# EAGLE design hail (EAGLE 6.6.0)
AUTHOR: Branden Ghena; REV: B; TITLE: Hail

## Sheet 1 of 4: Microcontroller
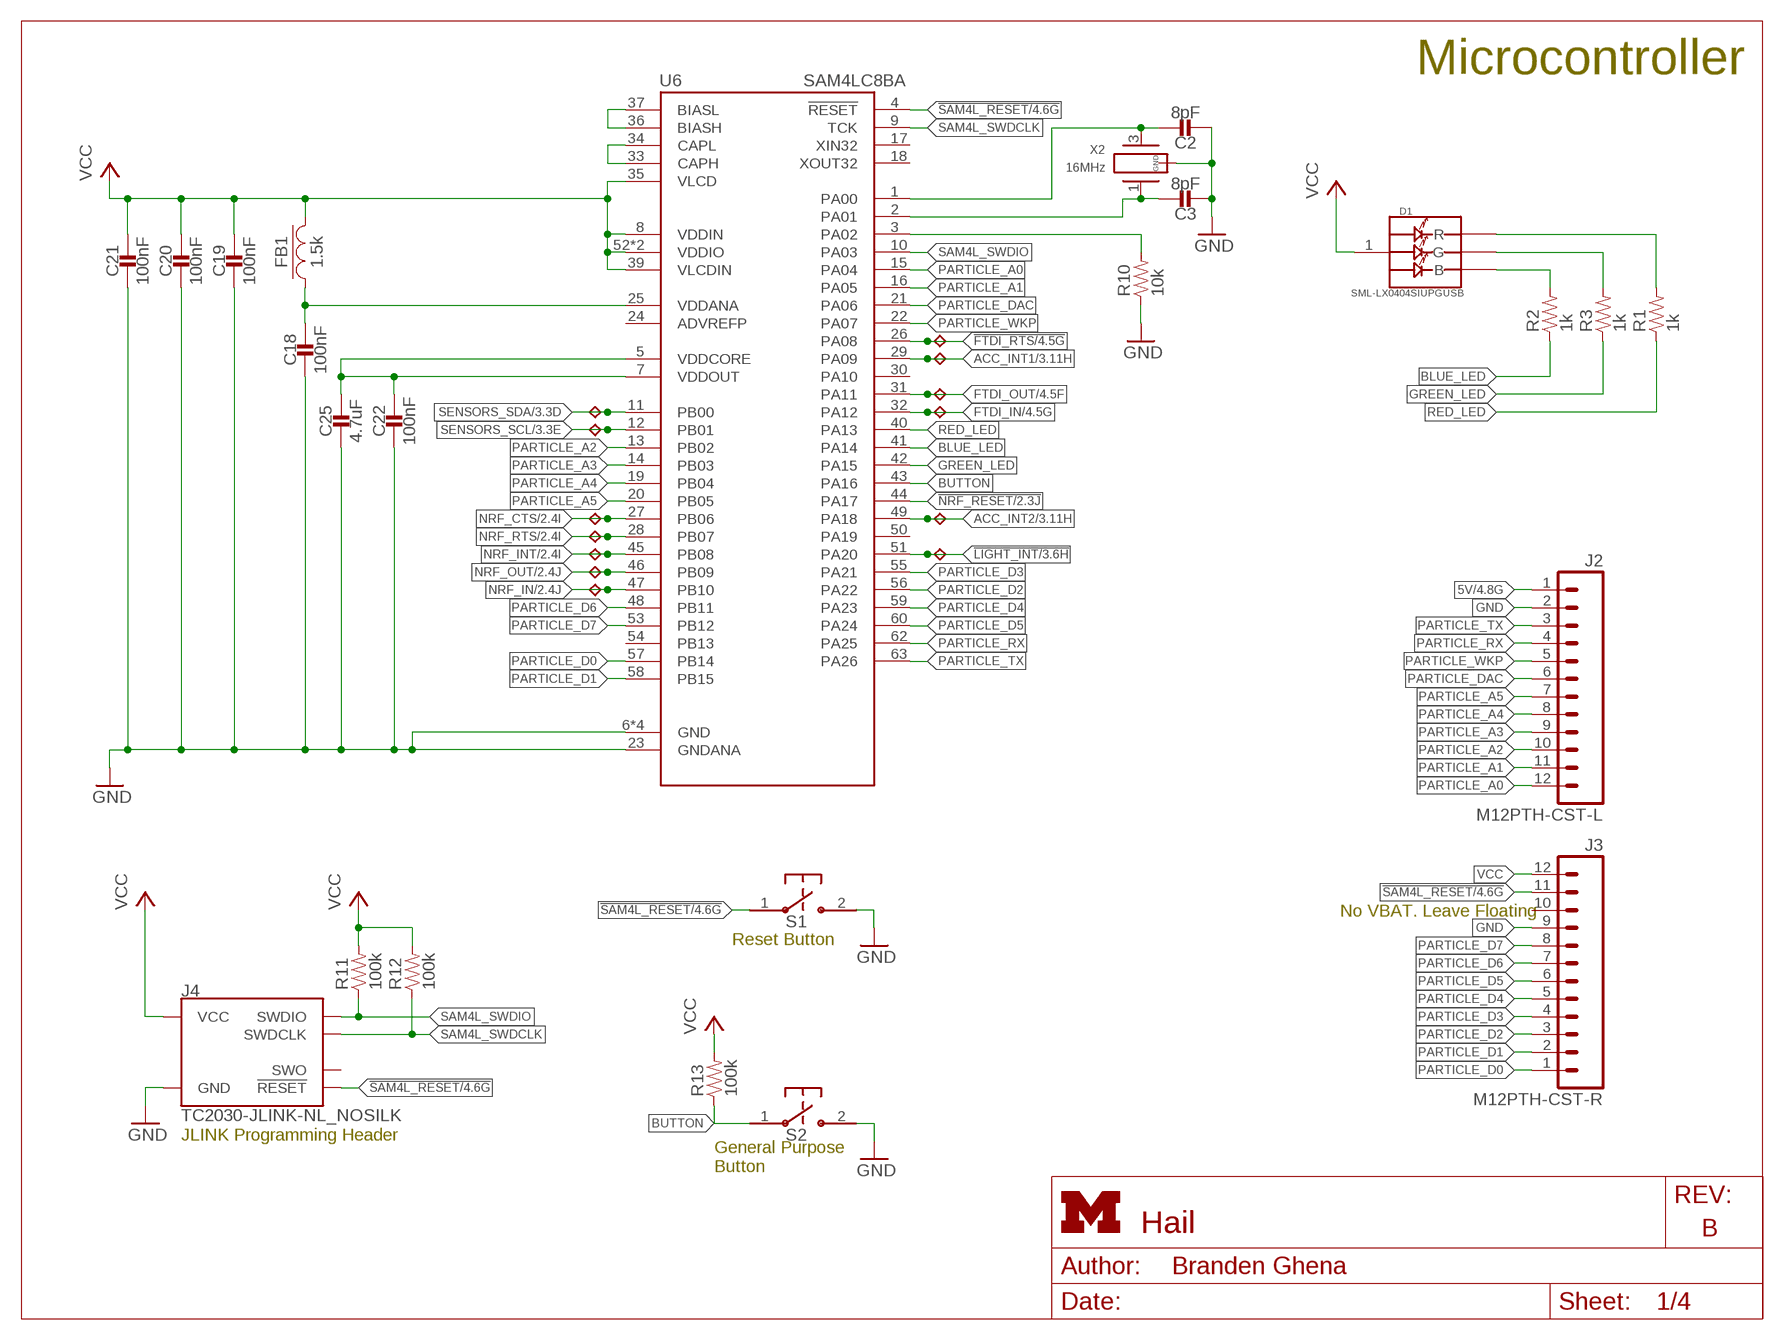
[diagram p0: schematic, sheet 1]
FRAME4 (LETTER_L_UMICH): HEIGHT: 8.5in; WIDTH: 11in
FRAME5 (LETTER_L_UMICH): HEIGHT: 8.5in; WIDTH: 11in

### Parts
C2  8pF  CAPACITOR0402_CAP  [0402_CAP]
C3  8pF  CAPACITOR0402_CAP  [0402_CAP]
C18  100nF  CAPACITOR0402_CAP  [0402_CAP]
C19  100nF  CAPACITOR0402_CAP  [0402_CAP]
C20  100nF  CAPACITOR0402_CAP  [0402_CAP]
C21  100nF  CAPACITOR0402_CAP  [0402_CAP]
C22  100nF  CAPACITOR0402_CAP  [0402_CAP]
C25  4.7uF  CAPACITOR0402_CAP  [0402_CAP]
D1  SML-LX0404SIUPGUSB  [1MM_SQ_4PAD]
FB1  1.5k  FERRITE_BEAD0402  [0402_CAP]
J2  M12PTH-CST-L  [1X12-CASTELLATED]
J3  M12PTH-CST-R  [1X12-CASTELLATED]
J4  TC2030-JLINK-NL_NOSILK  [TC2030-IDC-NL_NOSILK]
R1  1k  RESISTOR0402_RES  [0402_RES]
R2  1k  RESISTOR0402_RES  [0402_RES]
R3  1k  RESISTOR0402_RES  [0402_RES]
R10  10k  RESISTOR0402_RES  [0402_RES]
R11  100k  RESISTOR0402_RES  [0402_RES]
R12  100k  RESISTOR0402_RES  [0402_RES]
R13  100k  RESISTOR0402_RES  [0402_RES]
S1  B3U-1000P  [B3U-1000P]
S2  B3U-1000P  [B3U-1000P]
TP1  TPB1,27  [B1,27]
TP2  TPB1,27  [B1,27]
TP3  TPB1,27  [B1,27]
TP4  TPB1,27  [B1,27]
TP5  TPB1,27  [B1,27]
TP6  TPB1,27  [B1,27]
TP7  TPB1,27  [B1,27]
TP8  TPB1,27  [B1,27]
TP9  TPB1,27  [B1,27]
TP10  TPB1,27  [B1,27]
TP11  TPB1,27  [B1,27]
TP12  TPB1,27  [B1,27]
TP13  TPB1,27  [B1,27]
U6  SAM4LC8BA  [QFN-64-9MM]
X2  16MHz  FH1600015  [FHXXX]

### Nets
5V: J2.1 ; also sheet 4
!FTDI_RTS: TP11.TP U6.26(PA08) ; also sheet 4
!LIGHT_INT: TP10.TP U6.51(PA20) ; also sheet 3
!NRF_RESET: U6.44(PA17) ; also sheet 2
!SAM4L_RESET: J3.11 J4.3(!RESET) S1.1 U6.4(!RESET) ; also sheet 4
ACC_INT1: TP8.TP U6.29(PA09) ; also sheet 3
ACC_INT2: TP9.TP U6.49(PA18) ; also sheet 3
BLUE_LED: R2.1 U6.41(PA14)
BUCK/LDO_N1: R10.2 U6.3(PA02)
BUTTON: R13.1 S2.1 U6.43(PA16)
FTDI_IN: TP13.TP U6.32(PA12) ; also sheet 4
FTDI_OUT: TP12.TP U6.31(PA11) ; also sheet 4
GND: C2.2 C3.2 C18.2 C19.2 C20.2 C21.2 C22.2 C25.2 J2.2 J3.9 J4.5(GND) R10.1 S1.2 S2.2 U6.6(GND) U6.23(GNDANA) U6.38(GND) U6.64(GND) U6.GND X2.2(GND) X2.4(GND) ; also sheet 2,3,4
GREEN_LED: R3.1 U6.42(PA15)
N$7: D1.3(B) R2.2
N$8: D1.4(G) R3.2
N$9: D1.2(R) R1.2
N$15: U6.36(BIASH) U6.37(BIASL)
N$18: U6.33(CAPH) U6.34(CAPL)
N$20: C18.1 FB1.1 U6.25(VDDANA)
N$22: C22.1 C25.1 U6.5(VDDCORE) U6.7(VDDOUT)
NRF_CTS: TP1.TP U6.27(PB06) ; also sheet 2
NRF_IN: TP5.TP U6.47(PB10) ; also sheet 2
NRF_INT: TP3.TP U6.45(PB08) ; also sheet 2
NRF_OUT: TP4.TP U6.46(PB09) ; also sheet 2
NRF_RTS: TP2.TP U6.28(PB07) ; also sheet 2
PARTICLE_A0: J2.12 U6.15(PA04)
PARTICLE_A1: J2.11 U6.16(PA05)
PARTICLE_A2: J2.10 U6.13(PB02)
PARTICLE_A3: J2.9 U6.14(PB03)
PARTICLE_A4: J2.8 U6.19(PB04)
PARTICLE_A5: J2.7 U6.20(PB05)
PARTICLE_D0: J3.1 U6.57(PB14)
PARTICLE_D1: J3.2 U6.58(PB15)
PARTICLE_D2: J3.3 U6.56(PA22)
PARTICLE_D3: J3.4 U6.55(PA21)
PARTICLE_D4: J3.5 U6.59(PA23)
PARTICLE_D5: J3.6 U6.60(PA24)
PARTICLE_D6: J3.7 U6.48(PB11)
PARTICLE_D7: J3.8 U6.53(PB12)
PARTICLE_DAC: J2.6 U6.21(PA06)
PARTICLE_RX: J2.4 U6.62(PA25)
PARTICLE_TX: J2.3 U6.63(PA26)
PARTICLE_WKP: J2.5 U6.22(PA07)
RED_LED: R1.1 U6.40(PA13)
SAM4L_SWDCLK: J4.4(SWDCLK) R12.1 U6.9(TCK)
SAM4L_SWDIO: J4.2(SWDIO) R11.1 U6.10(PA03)
SAM4L_XIN1: C2.1 U6.1(PA00) X2.3
SAM4L_XOUT1: C3.1 U6.2(PA01) X2.1
SENSORS_SCL: TP7.TP U6.12(PB01) ; also sheet 3
SENSORS_SDA: TP6.TP U6.11(PB00) ; also sheet 3
VCC: C19.1 C20.1 C21.1 D1.1(VDD) FB1.2 J3.12 J4.1(VCC) R11.2 R12.2 R13.2 U6.8(VDDIN) U6.35(VLCD) U6.39(VLCDIN) U6.52(VDDIO) U6.61(VDDIO) ; also sheet 2,3,4
Unconnected: J3.10 J4.6(SWO) U6.17(XIN32) U6.18(XOUT32) U6.30(PA10) U6.50(PA19) U6.54(PB13)

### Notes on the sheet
- Microcontroller
- No VBAT. Leave Floating
- Reset Button
- JLINK Programming Header
- General Purpose
  Button

## Sheet 2 of 4: BLE Radio
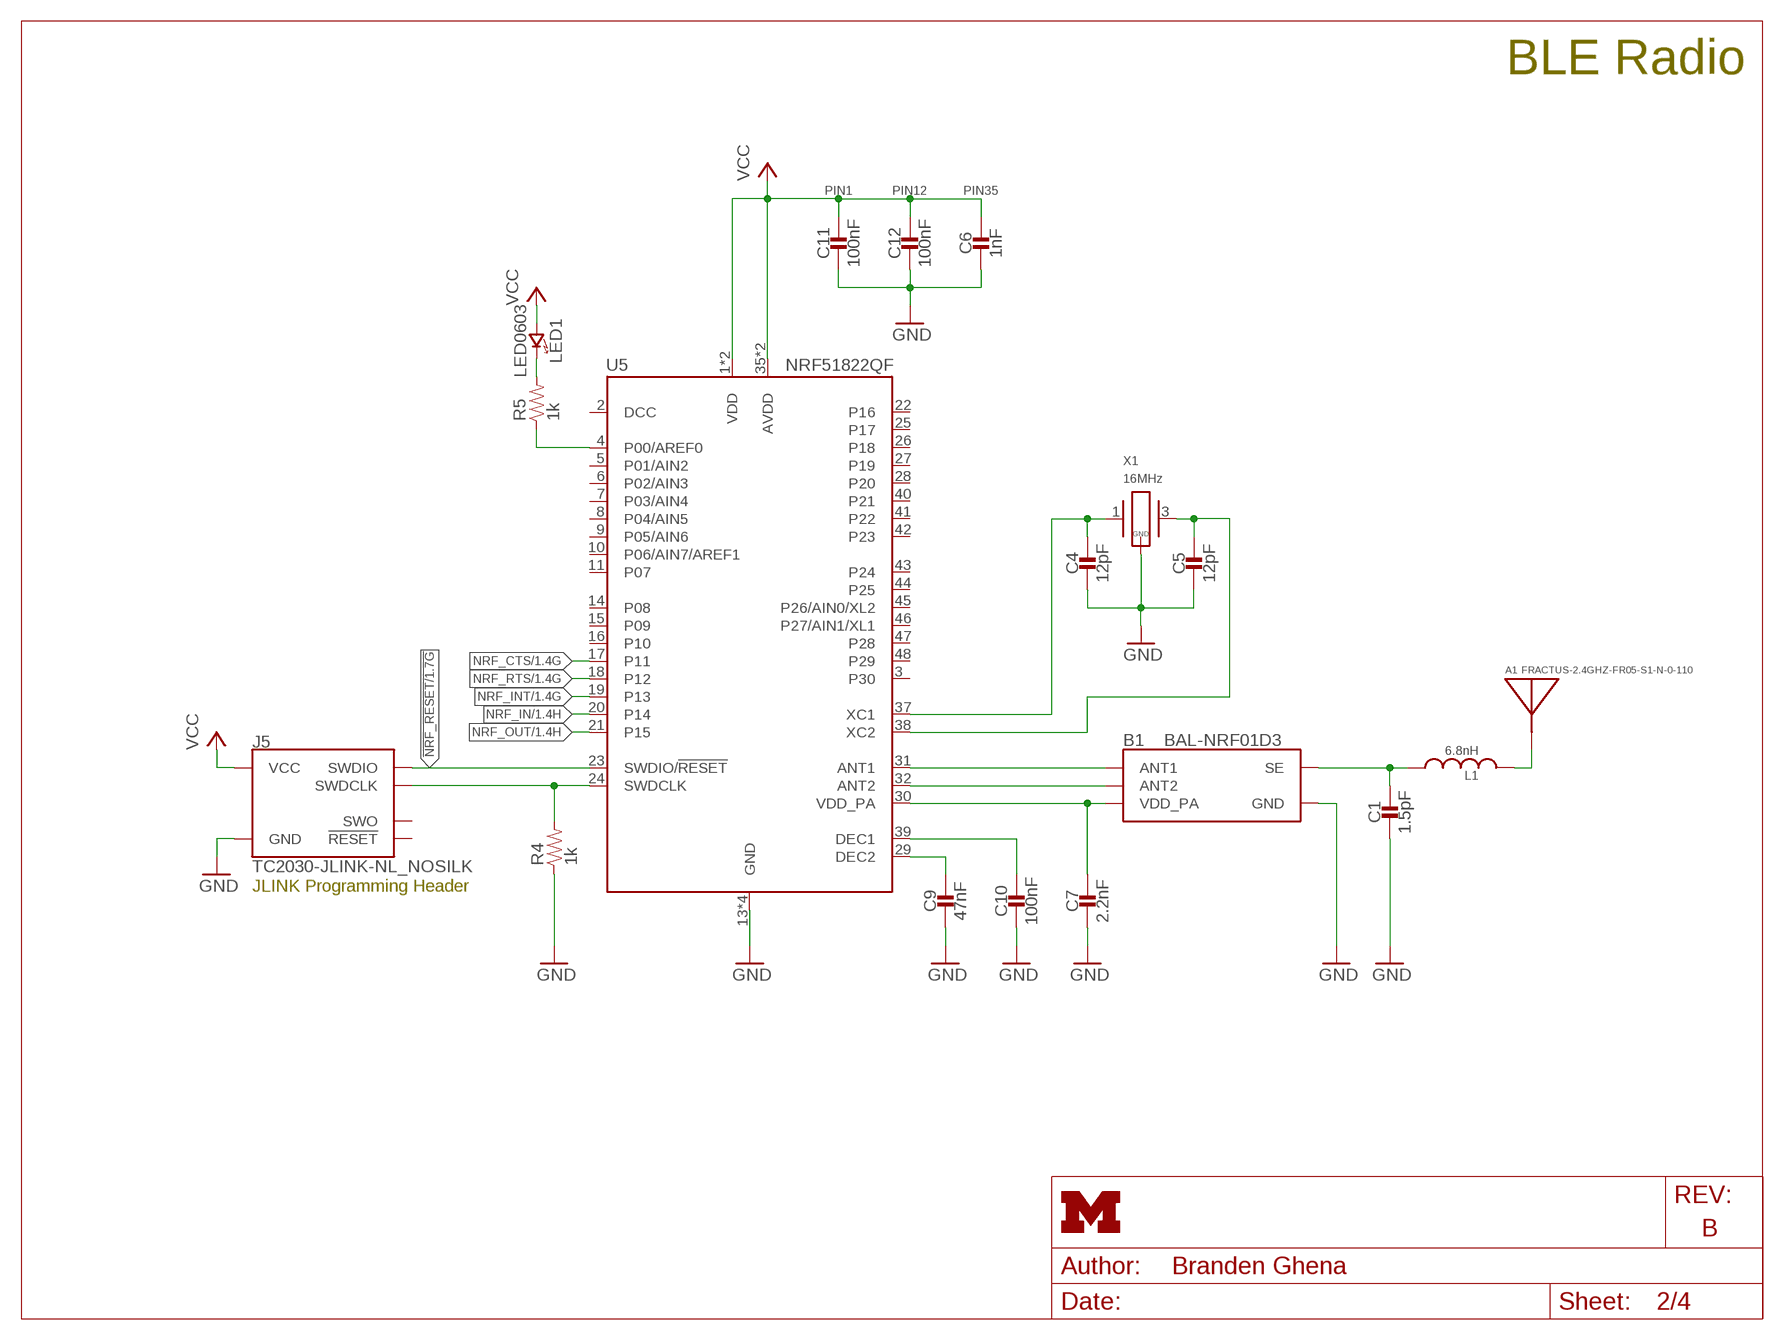
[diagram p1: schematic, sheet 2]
FRAME2 (LETTER_L_UMICH): HEIGHT: 8.5in; WIDTH: 11in
FRAME3 (LETTER_L_UMICH): HEIGHT: 8.5in; TITLE: Hail; WIDTH: 11in

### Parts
A1  FRACTUS-2.4GHZ-FR05-S1-N-0-110  [FRACTUS-ANTENNA-FR05-S1-N-0-110]
B1  BAL-NRF01D3  [BAL-NRF01D3]
C1  1.5pF  CAPACITOR0402_CAP  [0402_CAP]
C4  12pF  CAPACITOR0402_CAP  [0402_CAP]
C5  12pF  CAPACITOR0402_CAP  [0402_CAP]
C6  1nF  CAPACITOR0402_CAP  [0402_CAP]
C7  2.2nF  CAPACITOR0402_CAP  [0402_CAP]
C9  47nF  CAPACITOR0402_CAP  [0402_CAP]
C10  100nF  CAPACITOR0402_CAP  [0402_CAP]
C11  100nF  CAPACITOR0402_CAP  [0402_CAP]
C12  100nF  CAPACITOR0402_CAP  [0402_CAP]
J5  TC2030-JLINK-NL_NOSILK  [TC2030-IDC-NL_NOSILK]
L1  6.8nH  INDUCTOR0402  [0402_CAP]
LED1  LED0603  [LED-0603]
R4  1k  RESISTOR0402_RES  [0402_RES]
R5  1k  RESISTOR0402_RES  [0402_RES]
U5  NRF51822QF  [QFN-48-6MM]
X1  16MHz  TXC-8Y  [TXC-8Y]

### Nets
!NRF_RESET: J5.2(SWDIO) U5.23(SWDIO/!RESET) ; also sheet 1
GND: B1.GND C1.2 C4.2 C5.2 C6.2 C7.2 C9.2 C10.2 C11.2 C12.2 J5.5(GND) R4.1 U5.13(GND) U5.33(GND) U5.34(GND) U5.GND X1.2(GND) X1.4(GND) ; also sheet 1,3,4
N$3: C10.1 U5.39(DEC1)
N$4: C9.1 U5.29(DEC2)
N$6: J5.4(SWDCLK) R4.2 U5.24(SWDCLK)
N$10: R5.1 U5.4(P00/AREF0)
N$11: LED1.C(CATHODE) R5.2
N$12: B1.ANT1 U5.31(ANT1)
N$13: B1.VCC(VDD_PA) C7.1 U5.30(VDD_PA)
N$14: B1.ANT2 U5.32(ANT2)
N$16: C4.1 U5.37(XC1) X1.1
N$17: C5.1 U5.38(XC2) X1.3
N$19: B1.SE C1.1 L1.1
N$21: A1.ANT(ANTENNA) L1.2
NRF_CTS: U5.17(P11) ; also sheet 1
NRF_IN: U5.20(P14) ; also sheet 1
NRF_INT: U5.19(P13) ; also sheet 1
NRF_OUT: U5.21(P15) ; also sheet 1
NRF_RTS: U5.18(P12) ; also sheet 1
VCC: C6.1 C11.1 C12.1 J5.1(VCC) LED1.A(ANODE) U5.1(VDD) U5.12(VDD) U5.35(AVDD) U5.36(AVDD) ; also sheet 1,3,4
Unconnected: J5.3(!RESET) J5.6(SWO) U5.2(DCC) U5.3(P30) U5.5(P01/AIN2) U5.6(P02/AIN3) U5.7(P03/AIN4) U5.8(P04/AIN5) U5.9(P05/AIN6) U5.10(P06/AIN7/AREF1) U5.11(P07) U5.14(P08) U5.15(P09) U5.16(P10) U5.22(P16) U5.25(P17) U5.26(P18) U5.27(P19) U5.28(P20) U5.40(P21) U5.41(P22) U5.42(P23) U5.43(P24) U5.44(P25) U5.45(P26/AIN0/XL2) U5.46(P27/AIN1/XL1) U5.47(P28) U5.48(P29)

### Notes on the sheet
- BLE Radio
- PIN1 | PIN12 | PIN35
- JLINK Programming Header

## Sheet 3 of 4: Sensors
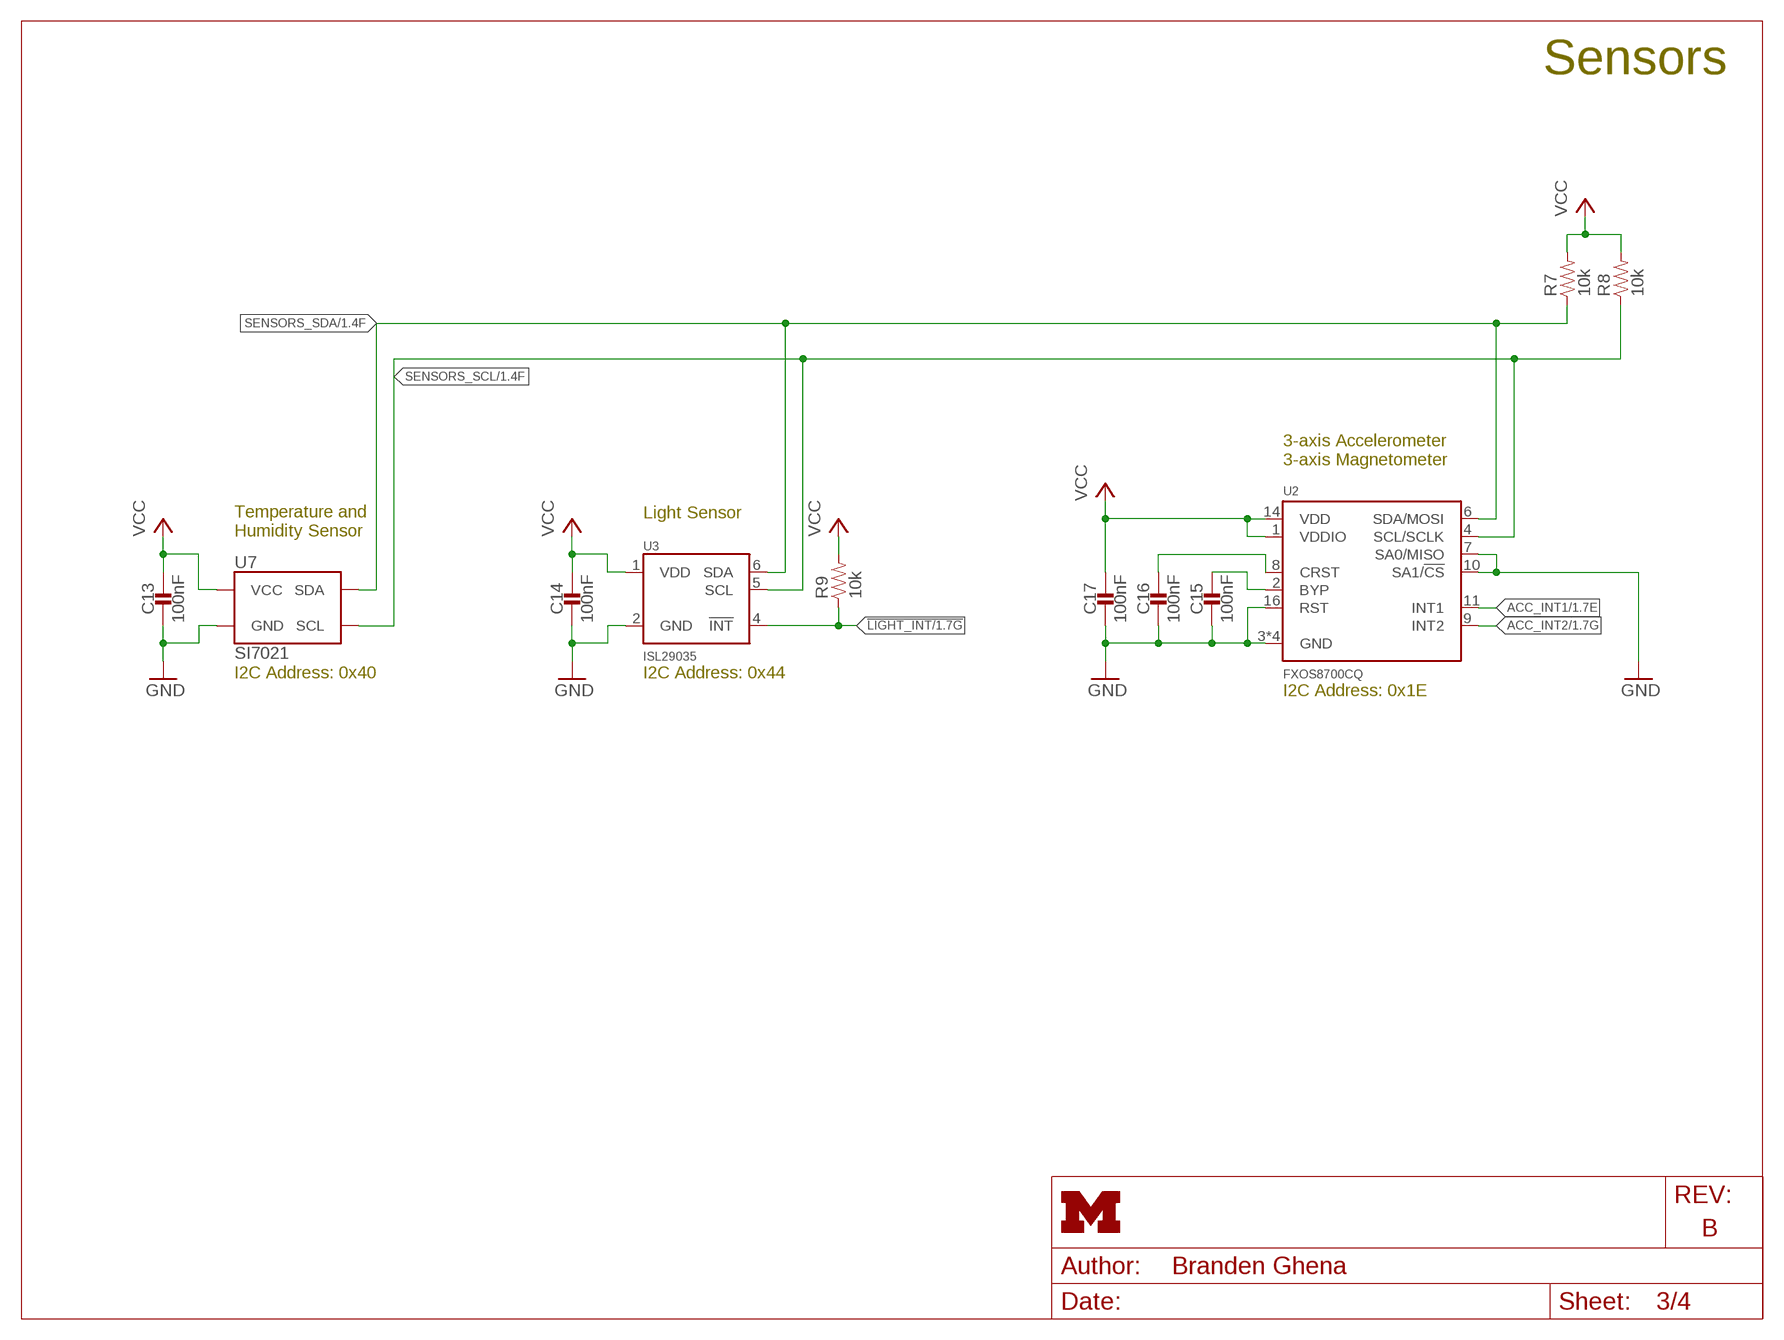
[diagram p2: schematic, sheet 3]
FRAME6 (LETTER_L_UMICH): HEIGHT: 8.5in; TITLE: Hail; WIDTH: 11in

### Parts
C13  100nF  CAPACITOR0402_CAP  [0402_CAP]
C14  100nF  CAPACITOR0402_CAP  [0402_CAP]
C15  100nF  CAPACITOR0402_CAP  [0402_CAP]
C16  100nF  CAPACITOR0402_CAP  [0402_CAP]
C17  100nF  CAPACITOR0402_CAP  [0402_CAP]
R7  10k  RESISTOR0402_RES  [0402_RES]
R8  10k  RESISTOR0402_RES  [0402_RES]
R9  10k  RESISTOR0402_RES  [0402_RES]
U2  FXOS8700CQ  [QFN-16-3MM]
U3  ISL29035  [ODFN-6-1.5MMX1.6MM]
U7  SI7021  [DFN-6/3MM]

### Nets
!LIGHT_INT: R9.1 U3.4(!INT) ; also sheet 1
ACC_INT1: U2.11(INT1) ; also sheet 1
ACC_INT2: U2.9(INT2) ; also sheet 1
GND: C13.2 C14.2 C15.2 C16.2 C17.2 U2.3(GND) U2.5(GND) U2.7(SA0/MISO) U2.10(SA1/!CS) U2.12(GND) U2.13(GND) U2.16(RST) U3.2(GND) U7.2(GND) ; also sheet 1,2,4
N$26: C15.1 U2.2(BYP)
N$27: C16.1 U2.8(CRST)
SENSORS_SCL: R8.1 U2.4(SCL/SCLK) U3.5(SCL) U7.6(SCL) ; also sheet 1
SENSORS_SDA: R7.1 U2.6(SDA/MOSI) U3.6(SDA) U7.1(SDA) ; also sheet 1
VCC: C13.1 C14.1 C17.1 R7.2 R8.2 R9.2 U2.1(VDDIO) U2.14(VDD) U3.1(VDD) U7.5(VCC) ; also sheet 1,2,4

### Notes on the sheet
- Sensors
- 3-axis Accelerometer
  3-axis Magnetometer
- Light Sensor
- Temperature and
  Humidity Sensor
- I2C Address: 0x40 | I2C Address: 0x44
- I2C Address: 0x1E

## Sheet 4 of 4: Power and USB
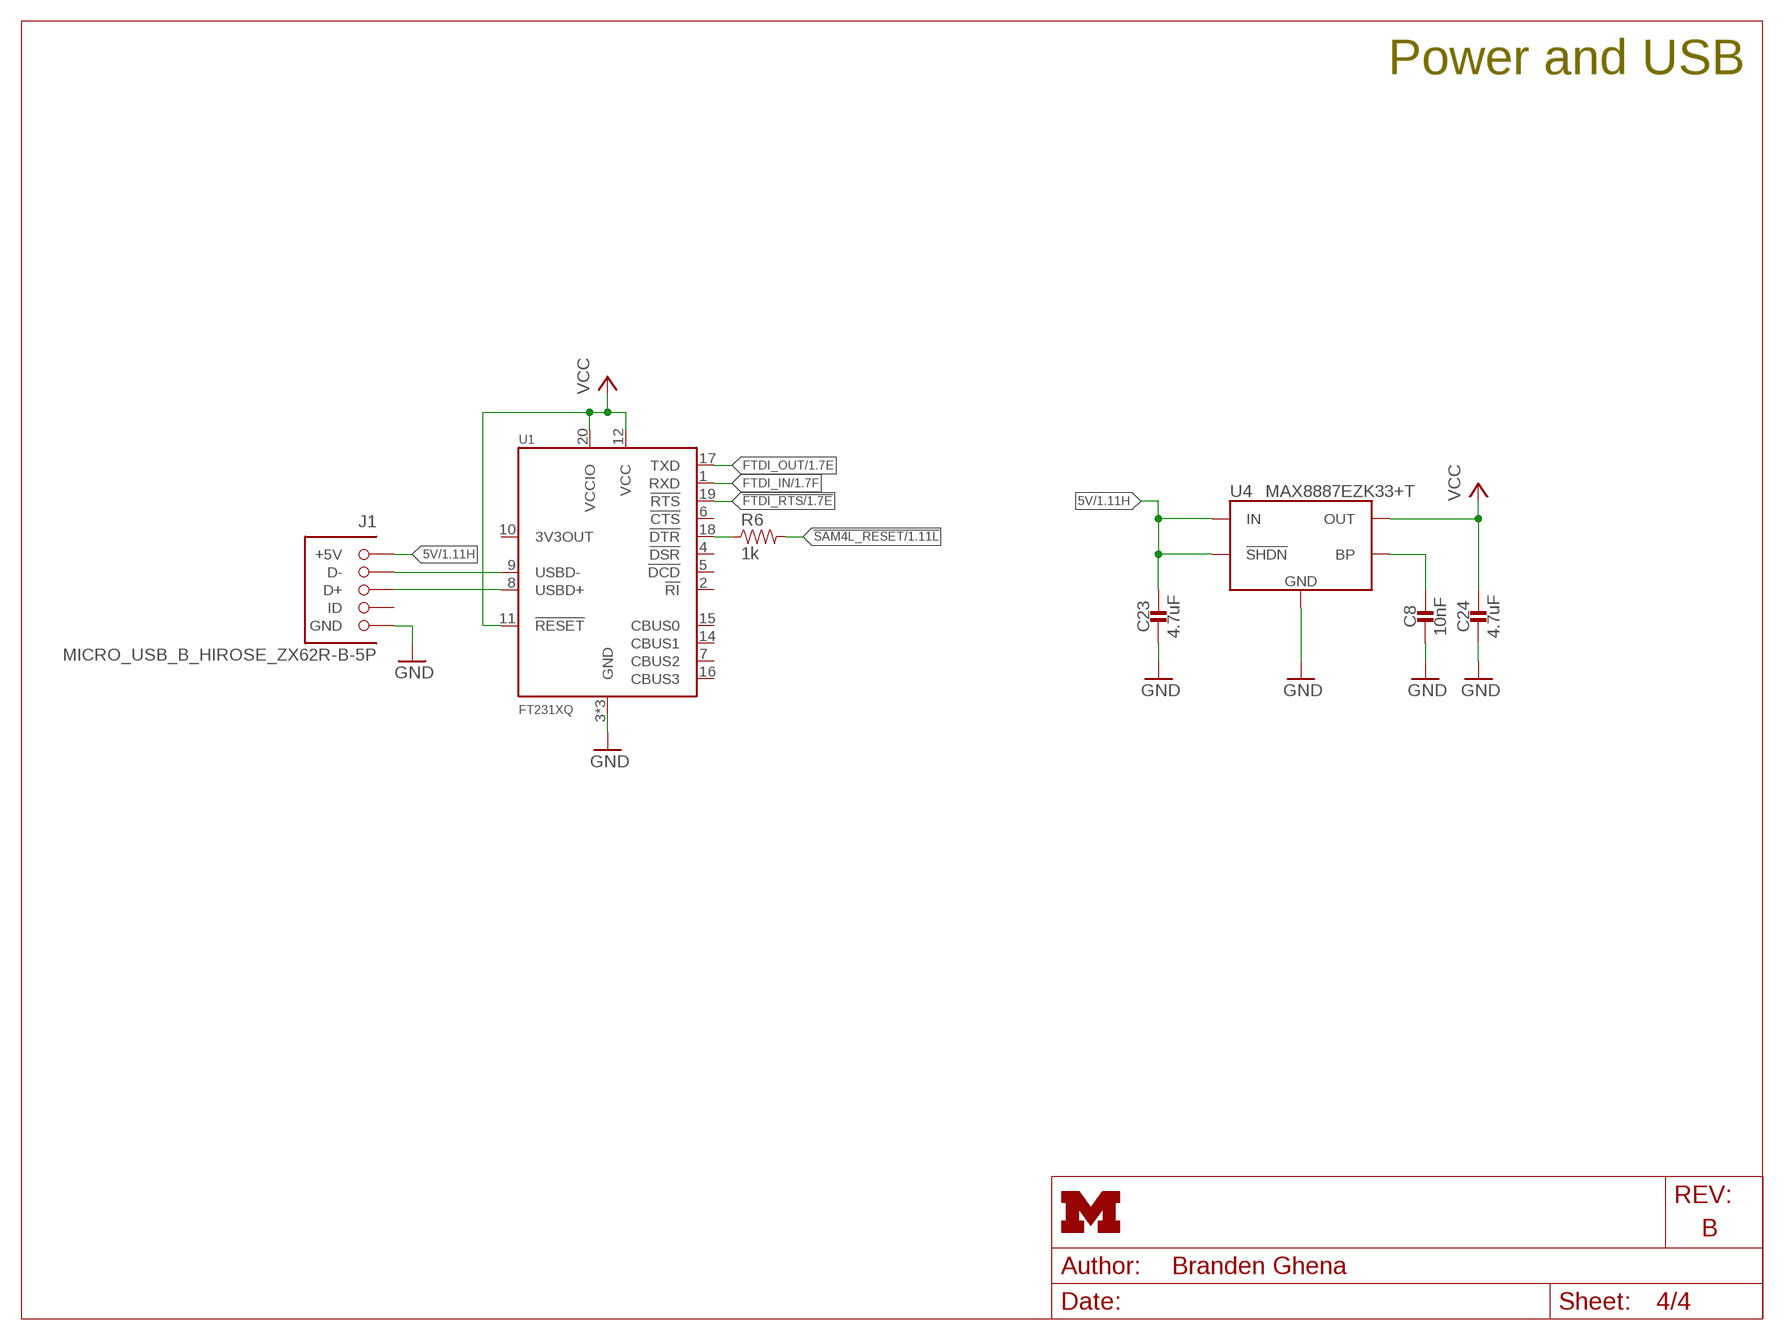
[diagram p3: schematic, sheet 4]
FRAME1 (LETTER_L_UMICH): HEIGHT: 8.5in; TITLE: Hail; WIDTH: 11in

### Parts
C8  10nF  CAPACITOR0402_CAP  [0402_CAP]
C23  4.7uF  CAPACITOR0402_CAP  [0402_CAP]
C24  4.7uF  CAPACITOR0402_CAP  [0402_CAP]
J1  MICRO_USB_B_HIROSE_ZX62R-B-5P  [USB_MICRO_B-HIROSE-ZX62R-B-5P]
R6  1k  RESISTOR0402_RES  [0402_RES]
U1  FT231XQ  [QFN-20-4MM]
U4  MAX8887EZK33+T  [SOT-23-5]

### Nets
5V: C23.1 J1.1(+5V) U4.1(IN) U4.3(!SHDN) ; also sheet 1
!FTDI_RTS: U1.19(!RTS) ; also sheet 1
!SAM4L_RESET: R6.2 ; also sheet 1
FTDI_IN: U1.1(RXD) ; also sheet 1
FTDI_OUT: U1.17(TXD) ; also sheet 1
GND: C8.2 C23.2 C24.2 J1.5(GND) U1.3(GND) U1.13(GND) U1.GND U4.2(GND) ; also sheet 1,2,3
N$1: J1.2(D-) U1.9(USBD-)
N$2: J1.3(D+) U1.8(USBD+)
N$5: C8.1 U4.4(BP)
N$24: R6.1 U1.18(!DTR)
VCC: C24.1 U1.11(!RESET) U1.12(VCC) U1.20(VCCIO) U4.5(OUT) ; also sheet 1,2,3
Unconnected: J1.4(ID) U1.2(!RI) U1.4(!DSR) U1.5(!DCD) U1.6(!CTS) U1.7(CBUS2) U1.10(3V3OUT) U1.14(CBUS1) U1.15(CBUS0) U1.16(CBUS3)

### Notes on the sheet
- Power and USB

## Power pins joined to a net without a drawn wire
ADVREFP: U6.24(ADVREFP)

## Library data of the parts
A1 = chips:FRACTUS-2.4GHZ-FR05-S1-N-0-110: Fractus Micro Reach Xtend; RICHARDSON_RFPD: FR05-S1-N-0110B
B1 = chips:BAL-NRF01D3: 50 ohm nominal input / conjugate match balun to nRF51422-QFAA, nRF24LE1, nRF51822-QFAA/AB, with integrated harmonic filter; DIGIKEY: 497-13637-1-ND; MOUSER: 511-BAL-NRF01D3
C1 = passives:CAPACITOR: 0402 Capacitor; DIGIKEY: 490-6212-1-ND
C2 C3 = passives:CAPACITOR: 0402 Capacitor; DIGIKEY: 490-8230-1-ND
C4 C5 = passives:CAPACITOR: 0402 Capacitor; DIGIKEY: 490-6197-1-ND
C6 = passives:CAPACITOR: 0402 Capacitor; DIGIKEY: 490-1303-1-ND
C7 = passives:CAPACITOR: 0402 Capacitor; DIGIKEY: 490-5419-1-ND
C8 = passives:CAPACITOR: 0402 Capacitor; DIGIKEY: 490-7763-1-ND
C9 = passives:CAPACITOR: 0402 Capacitor; DIGIKEY: 445-1264-1-ND
C10-C22 = passives:CAPACITOR: 0402 Capacitor; DIGIKEY: 490-10777-1-ND
C23-C25 = passives:CAPACITOR: 0402 Capacitor; DIGIKEY: 490-13252-1-ND
D1 = leds:SML-LX0404SIUPGUSB: 1mm^2 RGB LED; DIGIKEY: 67-2125-1-ND
FB1 = passives:FERRITE_BEAD; DIGIKEY: 1276-6395-1-ND
J1 = connector:MICRO_USB_B_HIROSE_ZX62R-B-5P: USB Micro B Connector Rounded side is up.; DIGIKEY: H125274CT-ND
J2 J3 = Particle:M12: Header 12 Standard 12-pin 0.1" header. Use with straight break away headers (SKU : PRT-00116), right angle break away headers (PRT-00553), swiss pins (PRT-00743), machine pins (PRT-00117), and female headers (PRT-00115).; DIGIKEY: S1011E-12-ND
J4 J5 = connector:TC2030-JLINK
L1 = passives:INDUCTOR: A very specific inductor; DIGIKEY: 490-6840-1-ND
LED1 = leds:LED: LED; DIGIKEY: 160-1837-6-ND
R1-R6 = passives:RESISTOR: Resistor; DIGIKEY: 1276-3430-1-ND
R7-R10 = passives:RESISTOR: Resistor; DIGIKEY: 1276-3431-1-ND
R11-R13 = passives:RESISTOR: Resistor; DIGIKEY: 1276-3432-1-ND
S1 S2 = switches:B3U: Switch; DIGIKEY: SW1020CT-ND
TP1-TP13 = testpad:TP: Test pad
U1 = chips:FT231X: USB Bridge, USB to UART USB 2.0 UART Interface; DIGIKEY: 768-1128-1-ND; MPN: FT231XQ-R
U2 = chips:FXOS8700CQ: Accelerometer, Magnetometer, 3 Axis Sensor, I2C/SPI; DIGIKEY: FXOS8700CQR1CT-ND; MPN: FXOS8700CQR1
U3 = chips:ISL29035: Optical Sensor Ambient 550nm I2C; DIGIKEY: ISL29035IROZ-T7CT-ND; MPN: ISL29035IROZ-T7
U4 = chips:MAX8887: IC REG LDO 3.3V 0.3A TSOT23-5; DIGIKEY: MAX8887EZK33+TCT-ND
U5 = chips:NRF51822: Multiprotocol Bluetooth® 4.0 low energy/2.4 GHz RF SoC; DIGIKEY: 1490-1049-1-ND
U6 = chips:SAM4LC8BA: SAM4L Microcontroller. 64QFN Package. 512 Flash.; DIGIKEY: ATSAM4LC8BA-MURCT-ND
U7 = chips:SI7021: IC TEMP SENSOR RH 2% DFN; DIGIKEY: 336-3141-ND
X1 = crystals:TXC-8Y: 2mmx1.6mm SMD Crystal; DIGIKEY: 887-2003-1-ND
X2 = crystals:FH1600015: Pericom Type FH 16 MHz 2.5 x 2.0 mm; DIGIKEY: FH1600015CT-ND

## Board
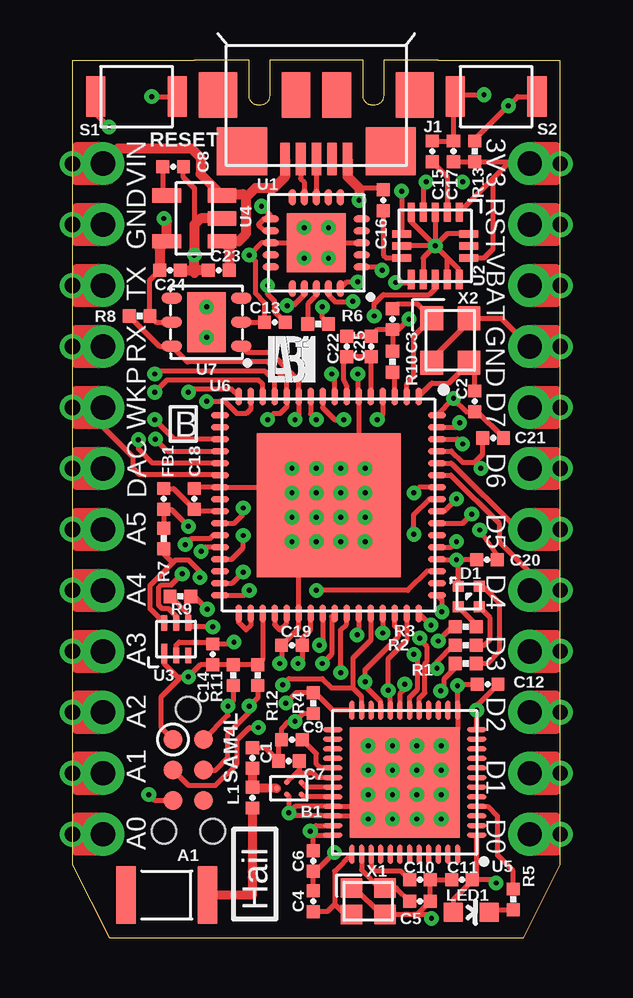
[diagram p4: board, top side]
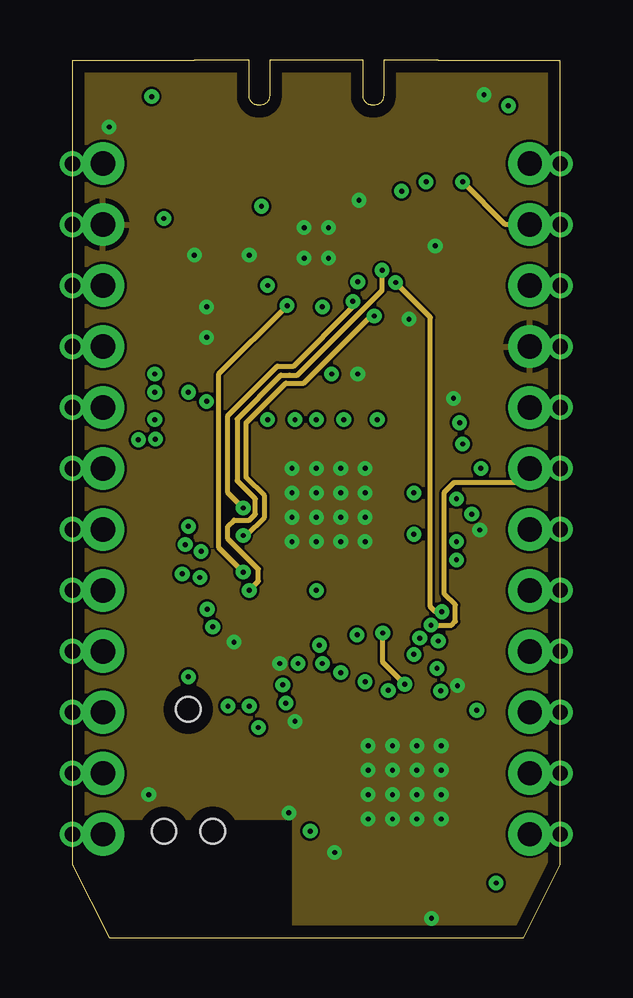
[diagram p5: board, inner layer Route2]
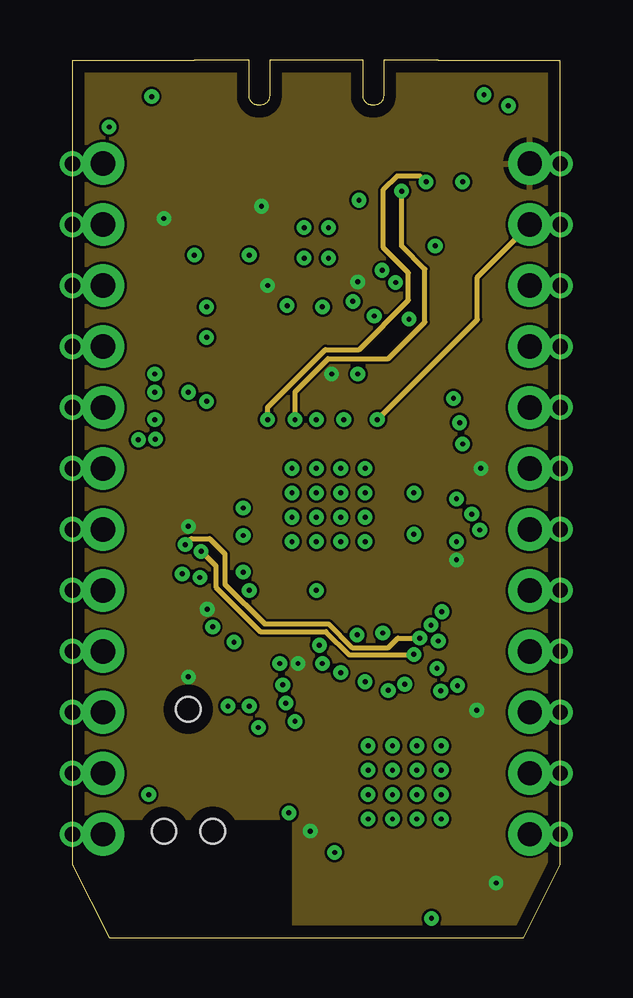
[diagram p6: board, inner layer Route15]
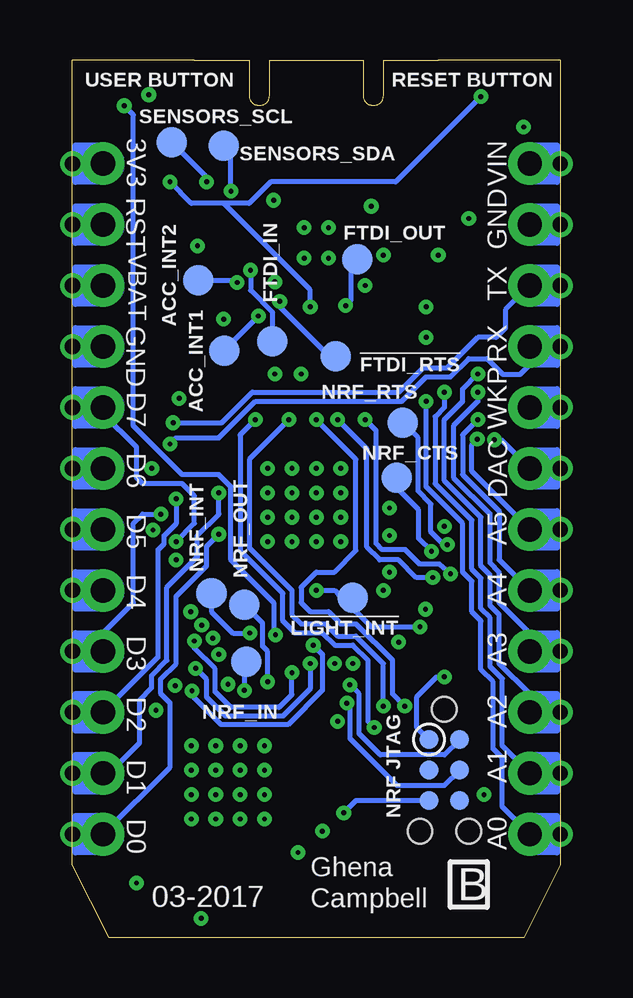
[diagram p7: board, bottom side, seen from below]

Size 20.32 x 36.58 mm. Coordinates in mm from the lower left corner, seen from the top.
Outline: 5.08,36.58 0,36.58 0,3.05 1.52,0 18.8,0 20.32,3.05 20.32,36.58 15.24,36.58
Copper layers (1+2*15+16): Top 0.0178mm / dielectric 12mil / Route2 0.0356mm / dielectric 28mil / Route15 0.0356mm / dielectric 12mil / Bottom 0.0178mm
Design rules "sunstone-4lyr_v1.0.0.3 *": minimum track width 4mil, minimum drill 8mil, track to track 4mil, track to pad 4mil, pad to pad 4mil, via to via 4mil, smd to smd 4mil, copper to edge 20mil, drill to drill 16mil, minimum pad ring 8mil, minimum via ring 8mil, stop-mask expansion 3mil, vias tented up to drill 50mil, thermal gap 8mil

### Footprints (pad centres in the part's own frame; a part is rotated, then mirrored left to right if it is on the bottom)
FRACTUS-ANTENNA-FR05-S1-N-0-110 = smd 0.8 x 2.4: ANT -1.7,0; NULL 1.7,0
BAL-NRF01D3 = smd 0.22 x 0.22: ANT1 -0.517,-0.25; ANT2 -0.517,0.25; GND 0.083,0.25; SE 0.516,0; VCC 0.083,-0.25
0402_CAP = smd 0.536 x 0.546: 1 -0.433,0; 2 0.433,0
1MM_SQ_4PAD = smd 0.457 x 0.457: 1 0.432,0.432; 2 0.432,-0.432; 3 -0.432,-0.432; 4 -0.432,0.432
USB_MICRO_B-HIROSE-ZX62R-B-5P = smd 0.4 x 1.35: 1 1.3,4.125; 2 0.65,4.125; 3 0,4.125; 4 -0.65,4.125; 5 -1.3,4.125 | smd 2.1 x 2: P$1 3.1,3.8; P$2 -3.1,3.8 | smd 1.6 x 1.9: P$3 -4.1,1.45; P$6 4.1,1.45 | smd 1.2 x 1.9: P$4 -0.85,1.45; P$5 0.85,1.45
1X12-CASTELLATED = drill 1.016 pad 1.778: 1 0,-13.97; 2 0,-11.43; 3 0,-8.89; 4 0,-6.35; 5 0,-3.81; 6 0,-1.27; 7 0,1.27; 8 0,3.81; 9 0,6.35; 10 0,8.89; 11 0,11.43; 12 0,13.97 | drill 0.635 pad 1.016: @1 1.27,-13.97; @2 1.27,-11.43; @3 1.27,-8.89; @4 1.27,-6.35; @5 1.27,-3.81; @6 1.27,-1.27; @7 1.27,1.27; @8 1.27,3.81; @9 1.27,6.35; @10 1.27,8.89; @11 1.27,11.43; @12 1.27,13.97
TC2030-IDC-NL_NOSILK = smd 0.787 x 0.787: 1 -1.27,-0.635; 2 -1.27,0.635; 3 0,-0.635; 4 0,0.635; 5 1.27,-0.635; 6 1.27,0.635 | hole 1.016: -2.54,0; 2.54,1.016; 2.54,-1.016
LED-0603 = smd 0.8 x 0.8: A 0,-0.75; C 0,0.75
0402_RES = smd 0.536 x 0.546: 1 -0.433,0; 2 0.433,0
B3U-1000P = smd 0.8 x 1.7: 1 -1.7,0; 2 1.7,0
B1,27 = smd 1.27 x 1.27: TP 0,0
QFN-20-4MM = smd 0.7 x 0.3: 1 -1.9,1; 2 -1.9,0.5; 3 -1.9,0; 4 -1.9,-0.5; 5 -1.9,-1; 11 1.9,-1; 12 1.9,-0.5; 13 1.9,0; 14 1.9,0.5; 15 1.9,1 | smd 0.3 x 0.7: 6 -1,-1.9; 7 -0.5,-1.9; 8 0,-1.9; 9 0.5,-1.9; 10 1,-1.9; 16 1,1.9; 17 0.5,1.9; 18 0,1.9; 19 -0.5,1.9; 20 -1,1.9 | smd 2.45 x 2.45: GND 0,0
QFN-16-3MM = smd 0.8 x 0.3: 1 -1.4,1; 2 -1.4,0.5; 3 -1.4,0; 4 -1.4,-0.5; 5 -1.4,-1; 9 1.4,-1; 10 1.4,-0.5; 11 1.4,0; 12 1.4,0.5; 13 1.4,1 | smd 0.3 x 0.8: 6 -0.5,-1.4; 7 0,-1.4; 8 0.5,-1.4; 14 0.5,1.4; 15 0,1.4; 16 -0.5,1.4
ODFN-6-1.5MMX1.6MM = smd 0.8 x 0.25: 1 -0.6,0.5 | smd 0.65 x 0.25: 2 -0.675,0; 3 -0.675,-0.5; 4 0.675,-0.5; 5 0.675,0; 6 0.675,0.5
SOT-23-5 = smd 0.6 x 1.2: 1 -0.95,-1.15; 2 0,-1.15; 3 0.95,-1.15; 4 0.95,1.15; 5 -0.95,1.15
QFN-48-6MM = smd 0.8 x 0.203: 1 -3,2.2; 2 -3,1.8; 3 -3,1.4; 4 -3,1; 5 -3,0.6; 6 -3,0.2; 7 -3,-0.2; 8 -3,-0.6; 9 -3,-1; 10 -3,-1.4; 11 -3,-1.8; 12 -3,-2.2; 25 3,-2.2; 26 3,-1.8; 27 3,-1.4; 28 3,-1; 29 3,-0.6; 30 3,-0.2; 31 3,0.2; 32 3,0.6; 33 3,1; 34 3,1.4; 35 3,1.8; 36 3,2.2 | smd 0.203 x 0.8: 13 -2.2,-3; 14 -1.8,-3; 15 -1.4,-3; 16 -1,-3; 17 -0.6,-3; 18 -0.2,-3; 19 0.2,-3; 20 0.6,-3; 21 1,-3; 22 1.4,-3; 23 1.8,-3; 24 2.2,-3; 37 2.2,3; 38 1.8,3; 39 1.4,3; 40 1,3; 41 0.6,3; 42 0.2,3; 43 -0.2,3; 44 -0.6,3; 45 -1,3; 46 -1.4,3; 47 -1.8,3; 48 -2.2,3 | smd 4.6 x 4.6: GND 0,0
QFN-64-9MM = smd 0.75 x 0.28: 1 -4.525,3.75; 2 -4.525,3.25; 3 -4.525,2.75; 4 -4.525,2.25; 5 -4.525,1.75; 6 -4.525,1.25; 7 -4.525,0.75; 8 -4.525,0.25; 9 -4.525,-0.25; 10 -4.525,-0.75; 11 -4.525,-1.25; 12 -4.525,-1.75; 13 -4.525,-2.25; 14 -4.525,-2.75; 15 -4.525,-3.25; 16 -4.525,-3.75; 33 4.525,-3.75; 34 4.525,-3.25; 35 4.525,-2.75; 36 4.525,-2.25; 37 4.525,-1.75; 38 4.525,-1.25; 39 4.525,-0.75; 40 4.525,-0.25; 41 4.525,0.25; 42 4.525,0.75; 43 4.525,1.25; 44 4.525,1.75; 45 4.525,2.25; 46 4.525,2.75; 47 4.525,3.25; 48 4.525,3.75 | smd 0.28 x 0.75: 17 -3.75,-4.525; 18 -3.25,-4.525; 19 -2.75,-4.525; 20 -2.25,-4.525; 21 -1.75,-4.525; 22 -1.25,-4.525; 23 -0.75,-4.525; 24 -0.25,-4.525; 25 0.25,-4.525; 26 0.75,-4.525; 27 1.25,-4.525; 28 1.75,-4.525; 29 2.25,-4.525; 30 2.75,-4.525; 31 3.25,-4.525; 32 3.75,-4.525; 49 3.75,4.525; 50 3.25,4.525; 51 2.75,4.525; 52 2.25,4.525; 53 1.75,4.525; 54 1.25,4.525; 55 0.75,4.525; 56 0.25,4.525; 57 -0.25,4.525; 58 -0.75,4.525; 59 -1.25,4.525; 60 -1.75,4.525; 61 -2.25,4.525; 62 -2.75,4.525; 63 -3.25,4.525; 64 -3.75,4.525 | smd 6 x 6: GND 0,0
DFN-6/3MM = smd 0.85 x 0.45: 1 -1.45,1; 2 -1.45,0; 3 -1.45,-1; 4 1.45,-1; 5 1.45,0; 6 1.45,1 | smd 1.6 x 2.5: P$1 0,0
TXC-8Y = smd 0.9 x 0.8: 1 -0.7,-0.55; 2 0.7,-0.55; 3 0.7,0.55; 4 -0.7,0.55
FHXXX = smd 1 x 0.95: 1 -0.925,-0.775; 2 0.925,-0.775; 3 0.925,0.775; 4 -0.925,0.775

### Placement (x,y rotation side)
A1  3.93,1.78 180 top
B1  9.02,6.22 180 top
C1  7.5,7.49 90 top
C2  16.76,22.35 270 top
C3  13.34,25.78 270 top
C4  10.03,1.52 90 top
C5  14.48,1.52 0 top
C6  10.03,3.2 270 top
C7  9.02,7.37 180 top
C8  4.19,32.13 0 top
C9  9.14,8.26 180 top
C10  14.48,2.41 0 top
C11  16.23,2.41 180 top
C12  17.3,10.57 180 top
C13  8.43,25.65 180 top
C14  5.84,11.81 90 top
C15  14.99,32.77 90 top
C16  12.95,30.73 90 top
C17  15.88,32.77 90 top
C18  5.08,18.29 90 top
C19  9.14,12.19 180 top
C20  17.27,15.75 0 top
C21  17.53,20.83 0 top
C22  11.43,24.64 90 top
C23  6.1,27.81 180 top
C24  4.06,27.81 0 top
C25  12.45,24.64 90 top
D1  16.51,14.22 90 top
FB1  3.81,18.29 270 top
J1  10.16,36.58 180 top
J2  1.27,18.29 180 top
J3  19.05,18.29 0 top
J4  4.83,6.99 270 top
J5  4.83,6.99 270 bottom
L1  7.5,5.84 270 top
LED1  16.61,1.07 270 top
R1  16.38,11.43 0 top
R2  16.38,12.19 0 top
R3  16.38,12.95 0 top
R4  10.03,9.78 90 top
R5  18.36,1.6 270 top
R6  10.24,25.58 0 top
R7  3.81,16.64 90 top
R8  2.79,25.91 0 top
R9  4.5,14.22 0 top
R10  13.34,24 270 top
R11  6.71,10.95 90 top
R12  7.72,10.95 90 top
R13  16.76,32.77 270 top
S1  2.67,35.05 180 top
S2  17.65,35.05 180 top
TP1  6.55,21.46 0 bottom
TP2  6.81,19.18 0 bottom
TP3  14.53,14.35 0 bottom
TP4  13.16,13.87 0 bottom
TP5  13.08,11.51 0 bottom
TP6  14.02,32.99 0 bottom
TP7  16.18,33.15 0 bottom
TP8  14,24.46 0 bottom
TP9  15.09,27.41 0 bottom
TP10  8.64,14.17 0 bottom
TP11  9.35,24.23 0 bottom
TP12  8.46,28.27 0 bottom
TP13  11.99,24.87 0 bottom
U1  10.16,28.96 180 top
U2  15.11,28.83 270 top
U3  4.32,12.45 90 top
U4  5.08,29.97 90 top
U5  13.84,6.48 180 top
U6  10.67,18.03 270 top
U7  5.59,25.65 180 top
U$1  [PHOTON-BOTTOM-SS]  0,0.51 0 top
U$2  [PHOTON-TOP-SS]  0,0.51 0 top
U$3  [LAB11_SOLID_80MIL]  8.13,23.11 0 top
X1  12.32,1.52 0 top
X2  15.75,24.89 270 top

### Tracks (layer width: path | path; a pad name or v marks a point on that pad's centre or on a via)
5V
  Top 0.203: U4.3 6.3,30.99
  Top 0.406: J1.1 8.86,31.72 8.38,31.24 7.62,31.24 7.24,30.86 | 7.24,30.86 7.24,29.34 6.92,29.02 U4.1 6.53,28.72 C23.1 | J2.1 1.91,32.89 4.95,32.89 5.33,32.51 5.33,31.82 U4.3 | 6.3,30.99 7.11,30.99 7.24,30.86
!FTDI_RTS  (via drill 0.2)
  Top 0.203: U6.26 6.74,17.28 7.11,17.65 v7.11,17.91 | U1.19 10.66,26.8 10.97,26.49 11.66,26.49 v11.68,26.52
  Route2 0.203: v7.11,17.91 6.48,18.54 6.48,21.76 8.54,23.82 9.22,23.82 11.68,26.29 v11.68,26.52
  Bottom 0.203: v11.68,26.52 11.68,26.29 9.63,24.23 TP11.TP
!LIGHT_INT  (via drill 0.2)
  Top 0.203: U6.51 14.78,15.28 13.97,14.48 v10.16,14.48 | v5.84,12.95 4.99,12.95 U3.4 4.82,13.47 R9.1
  Bottom 0.203: v10.16,14.48 9.4,14.48 9.22,14.3 9.09,14.17 | 9.09,14.17 7.87,12.95 v5.84,12.95 | TP10.TP 9.09,14.17
!NRF_RESET  (via drill 0.2)
  Top 0.203: v8.76,10.54 9.02,10.79 10.41,10.79 10.79,10.41 11.68,10.41 | U5.23 12.04,10.05 11.68,10.41 | U6.44 12.42,12.39 11.68,11.66 11.68,10.41
  Bottom 0.203: J5.2 4.83,7.62 7.5,7.62 8.38,8.51 8.38,10.16 v8.76,10.54
!SAM4L_RESET  (via drill 0.2)
  Top 0.203: 4.19,6.86 J4.3 4.83,6.35 5.95,6.35 6.86,7.25 6.86,8.26 7.37,8.76 v7.75,8.76 | U6.4 12.92,21.81 v12.7,21.59 | v3.3,35.05 S1.1 | R6.2 10.41,25.83 v10.41,26.29
  Route2 0.203: J3.11 18.03,29.72 v16.26,31.5
  Route15 0.203: J3.11 16.87,27.53 16.87,25.76 v12.7,21.59
  Bottom 0.203: v7.75,8.76 8,9.02 8,11.56 8.64,12.19 9.4,12.19 9.91,12.7 11.05,12.7 11.56,13.21 11.56,14.35 13.34,16.13 13.34,20.95 v12.7,21.59 | 14.02,30.6 12.96,30.6 12.06,31.5 6.86,31.5 v3.3,35.05 | 14.02,30.6 15.36,30.6 v16.26,31.5 | v10.41,26.29 10.41,27 14.02,30.6
ACC_INT1  (via drill 0.2)
  Top 0.203: U6.29 6.64,15.78 7.11,16.26 v7.11,16.76 | v12.57,25.91 12.57,26.42 12.95,26.8 14.86,26.8 15.11,27.05 U2.11
  Route2 0.203: v7.11,16.76 7.24,16.76 8,17.53 8,18.41 7.24,19.18 7.24,21.47 8.89,23.11 9.63,23.11 12.42,25.91 v12.57,25.91
  Bottom 0.203: TP8.TP 13.99,24.49 v12.57,25.91
ACC_INT2  (via drill 0.2)
  Top 0.203: v13.46,27.3 13.99,27.3 U2.9 | U6.49 15.39,14.09 v15.39,13.59
  Route2 0.203: v13.46,27.3 14.91,25.86 14.91,13.79 15.11,13.59 v15.39,13.59
  Bottom 0.203: TP9.TP 13.56,27.41 v13.46,27.3
BLUE_LED  (via drill 0.2)
  Top 0.203: U6.41 10.79,13.39 10.79,11.81 v10.41,11.43 | v15.19,11.23 15.19,11.51 15.88,12.19 R2.1
  Bottom 0.203: v10.41,11.43 10.41,10.38 11.55,9.24 13.94,9.24 14.73,10.03 14.73,10.77 v15.19,11.23
BUCK/LDO_N1
  Top 0.203: U6.3 13.42,23.74 R10.2
BUTTON  (via drill 0.2)
  Top 0.203: U6.43 11.92,12.68 v11.86,12.62 | S2.1 18.54,35.05 v18.16,34.67 16.76,33.27 R13.1
  Bottom 0.203: v11.86,12.62 11.94,12.7 11.94,13.97 13.72,15.75 13.72,18.8 14.22,19.3 15.75,19.3 17.78,21.34 17.78,34.29 v18.16,34.67
FTDI_IN  (via drill 0.2)
  Top 0.203: U6.32 7.17,14.28 v7.37,14.48 | U1.1 12.76,27.96 v12.9,27.81
  Route2 0.203: v7.37,14.48 7.75,14.86 7.75,15.37 6.48,16.64 6.48,17.14 6.73,17.4 7.37,17.4 7.62,17.65 7.62,18.29 6.86,19.05 6.86,21.61 8.69,23.44 9.04,23.44 9.37,23.44 12.9,26.98 v12.9,27.81
  Bottom 0.203: v12.9,27.81 12.9,26.98 11.99,26.06 TP13.TP
FTDI_OUT  (via drill 0.2)
  Top 0.203: U6.31 6.66,14.78 v7.11,15.24 | U1.17 9.66,26.8 9.2,26.34 v8.94,26.34
  Route2 0.203: v7.11,15.24 6.1,16.26 6.1,23.5 v8.94,26.34
  Bottom 0.203: v8.94,26.34 8.71,26.57 8.71,28.02 TP12.TP
GND  (via drill 0.2)
  Top 0.203: U1.3 U1.GND U1.13 7.87,28.96 v7.37,28.45 7.62,28.19 7.62,26.85 8,26.47 C13.2 U7.2 | C3.2 R10.1 | U6.GND 11.92,19.28 U6.6 11.89,22.59 v11.89,23.5 | U6.GND 9.92,18.78 U6.23 5.14,18.78 C18.2 | U6.GND 9.42,16.78 U6.38 9.4,13.49 9.4,12.88 C19.2 8.71,11.51 v8.64,11.43 | X2.2 14.97,24.12 16.52,25.67 X2.4 17.87,25.82 J3.9 19.05,24.2 | C22.2 C25.2 12.72,25.35 C3.2 | U6.64 15.88,22.47 | 15.88,22.47 v15.88,22.48 | 15.88,22.47 16.42,21.92 C2.2 16.87,21.92 C21.2 | U5.GND 12.84,5.48 U5.33 9.29,5.48 v9.02,5.21 | 9.14,5.08 v9.02,5.21 | U5.GND 12.44,5.08 U5.34 9.15,5.08 v9.02,5.21 | B1.GND 9.02,5.89 v9.02,5.21 | U5.GND 16.04,8.68 U5.13 v16.04,10.51 16.1,10.57 C12.2 | X1.4 11.77,2.07 12.87,0.97 X1.2 14.36,0.97 | R4.1 9.6,9.35 v9.27,9.02 9.02,9.02 8.71,8.71 C9.2 8.58,8.13 C7.2 8.02,7.93 C1.2 | 14.36,0.97 C5.2 C10.2 C11.2 | C20.2 17.7,15.95 v16.97,16.99 | C3.2 13.59,25.35 v14.02,25.78 | J4.5 3.43,5.71 v3.17,5.97 | U3.2 4.32,12.19 4.45,12.32 5.77,12.32 C14.2 6.66,12.24 v6.73,12.32 | 5.08,29.46 5.08,31.24 4.62,31.7 C8.2 | S1.2 0.97,34.34 v1.52,33.78 | U2.13 16.11,27.83 15.61,28.33 | 15.61,28.33 v15.11,28.83 | v15.11,28.83 U2.7 | U2.16 15.61,29.33 v15.11,28.83 | U2.3 v15.11,28.83 | U2.5 14.11,29.83 v15.11,28.83 | U2.12 15.61,28.33 | v15.11,28.83 14.61,28.33 U2.10 | C15.2 C17.2 15.88,34.97 S2.2 16.03,35.13 v17.14,35.13 | C16.2 12.88,31.24 11.94,31.24 | 14.36,0.97 14.8,0.97 v14.96,0.81 | C4.2 C6.2 10.13,2.77 v10.92,3.56
  Top 0.406: J1.5 11.46,31.72 11.94,31.24 v11.94,30.73 | U4.2 5.33,29.97 5.08,29.72 5.08,29.46 v5.08,28.45 5.08,27.94 | 5.08,27.94 5.08,27.71 5.19,27.81 C23.2 | C24.2 4.95,27.81 5.08,27.94
  Route2 0.203: v16.04,10.51
  Bottom 0.203: J5.5 8.51,5.71 v9.02,5.21
  other vias: 5.59,26.29 5.59,25.02 9.65,29.59 9.65,29.59 10.67,29.59 10.67,28.32 9.65,28.32 10.16,18.54 10.16,17.53 11.18,17.53 11.18,18.54 11.18,19.56 10.16,19.56 9.14,19.56 9.14,18.54 9.14,17.53 9.14,16.51 10.16,16.51 11.18,16.51 12.19,16.51 12.19,17.53 12.19,18.54 12.19,19.56 13.34,6.99 13.34,5.97 13.34,6.99 14.35,6.99 14.35,5.97 13.34,8 14.35,8 15.37,8 15.37,6.99 15.37,5.97 15.37,4.95 14.35,4.95 13.34,4.95 12.32,4.95 12.32,5.97 12.32,6.99 12.32,8
  pour Route2: 9.27,0 9.27,5 0,5 0,36.58 20.32,36.58 20.32,3.05 18.8,0
GREEN_LED  (via drill 0.2)
  Top 0.203: v11.18,11.05 11.18,12.83 11.42,13.07 U6.42 | 15.88,12.95 R3.1 15.82,12.95 v15.24,12.37
  Bottom 0.203: v15.24,12.37 15.24,12.06 14.38,11.2 14.38,10.25 13.73,9.6 11.71,9.6 11.18,10.13 v11.18,11.05
N$1
  Top 0.203: J1.2 9.51,31.64 9.65,31.5 U1.9
N$2
  Top 0.203: J1.3 U1.8
N$3
  Top 0.203: C10.1 13.65,2.79 12.57,2.79 12.44,2.92 U5.39
N$4
  Top 0.203: U5.29 10.32,7.08 10.16,7.24 10.16,7.67 C9.1
N$5
  Top 0.203: 3.81,31.04 U4.4 3.76,31.09 C8.1
N$6  (via drill 0.2)
  Top 0.203: v8.89,9.78 9.32,10.21 R4.2 10.11,10.21 10.84,9.48 U5.24
  Bottom 0.203: J5.4 4.83,6.35 6.8,6.35 8.76,8.31 8.76,9.65 v8.89,9.78
N$7
  Top 0.203: R2.2 17.14,12.19 17.4,12.45 17.4,13.34 D1.3
N$8
  Top 0.203: D1.4 16.82,13.05 R3.2
N$9
  Top 0.203: D1.2 17.09,14.66 17.78,13.97 17.78,11.94 17.27,11.43 R1.2
N$10
  Top 0.203: R5.1 18.36,2.79 17.7,3.45 17.7,5.07 17.3,5.48 U5.4
N$11
  Top 0.203: LED1.C 17.46,1.17 R5.2
N$12
  Top 0.203: U5.31 9.73,6.28 B1.ANT1
N$13
  Top 0.203: U5.30 10.21,6.68 10.03,6.86 9.32,6.86 | 9.32,6.86 B1.VCC | C7.1 9.45,6.99 9.32,6.86
N$14
  Top 0.203: U5.32 9.63,5.88 B1.ANT2
N$15
  Top 0.203: U6.36 8.42,13.04 8.64,12.83 8.92,13.11 U6.37
N$16
  Top 0.203: U5.37 11.62,3.48 10.92,2.77 10.92,1.4 | 11.6,0.97 X1.1 11.35,0.97 10.92,1.4 | 10.92,1.4 10.62,1.09 C4.1
N$17
  Top 0.203: U5.38 12.04,2.82 12.79,2.07 X1.3 13.49,2.07 C5.1
N$18
  Top 0.203: U6.34 7.42,13.01 7.24,12.83 6.92,13.15 U6.33
N$19
  Top 0.381: B1.SE 7.5,6.22 L1.1 C1.1
N$20
  Top 0.203: U6.25 5.15,17.78 C18.1 4.21,18.72 FB1.1
N$21
  Top 0.381: L1.2 7.5,1.78 A1.ANT
N$22
  Top 0.203: U6.5 12.42,23.98 C25.1 C22.1 11.3,23.95 11.3,23.24 11.42,23 U6.7 11.42,22.87
N$24
  Top 0.203: U1.18 10.16,26.77 9.8,26.41 R6.1
N$26
  Top 0.203: C15.1 15.61,31.71 U2.2
N$27
  Top 0.203: C16.1 12.95,28.45 13.07,28.33 U2.8
NRF_CTS  (via drill 0.2)
  Top 0.203: v4.7,16.38 4.95,16.64 5.71,16.64 5.86,16.78 U6.27 | U5.17 14.44,9.97 14.68,10.21 14.68,11.43 14.76,11.51 14.76,12.14 14.47,12.43 v14.47,12.49
  Route15 0.203: v4.7,16.38 4.95,16.64 5.71,16.64 6.35,16 6.35,14.73 8,13.08 10.67,13.08 11.65,12.1 13.16,12.1 13.55,12.49 v14.47,12.49
  Bottom 0.203: v4.7,16.38 4.85,16.38 5.38,16.92 5.38,18.09 5.92,18.62 5.92,20.83 TP1.TP
NRF_IN  (via drill 0.2)
  Top 0.203: U6.47 13.92,12.39 13.16,11.63 v13.16,10.31 13.24,10.23 U5.20
  Bottom 0.203: TP5.TP 13.16,11.43 v13.16,10.31
NRF_INT  (via drill 0.2)
  Top 0.203: U6.45 12.92,12.71 v12.93,12.7 | v13.84,10.57 13.84,10.36 13.64,10.16 U5.19
  Route2 0.203: v13.84,10.57 12.93,11.48 v12.93,12.7
  Bottom 0.203: TP3.TP 14.53,13.59 13.64,12.7 v12.93,12.7
NRF_OUT  (via drill 0.2)
  Top 0.203: U6.46 13.42,13 13.59,12.83 13.59,12.57 12.19,11.18 v12.19,10.67 12.19,10.49 12.84,9.84 U5.21 12.84,9.76
  Bottom 0.203: v12.19,10.67 12.19,11.94 12.39,12.14 12.39,13.11 TP4.TP
NRF_RTS  (via drill 0.2)
  Top 0.203: U6.28 5.54,16.28 v5.36,16.1 | U5.18 14.04,10.03 14.38,10.36 14.38,11.66 v14.22,11.81
  Route15 0.203: v5.36,16.1 5.97,15.49 5.97,14.61 7.82,12.76 10.55,12.76 11.53,11.79 14.2,11.79 v14.22,11.81
  Bottom 0.203: v5.36,16.1 5.89,16.64 5.89,17.83 6.81,18.75 TP2.TP
PARTICLE_A0  (via drill 0.2)
  Top 0.203: v5.59,22.35 6.35,22.35 6.86,21.84 7.24,21.84 7.42,22.02 U6.15
  Bottom 0.203: J2.12 2.41,5.46 2.41,7.49 2.79,7.87 2.79,10.67 3.3,11.18 3.3,13.21 3.68,13.59 3.68,14.86 4.06,15.24 4.06,17.27 5.59,18.8 v5.59,22.35
PARTICLE_A1  (via drill 0.2)
  Top 0.203: U6.16 6.62,22.86 4.95,22.86 v4.83,22.73
  Bottom 0.203: J2.11 2.41,8 2.41,10.79 2.92,11.3 2.92,13.34 3.3,13.72 3.3,14.99 3.68,15.37 3.68,17.4 5.21,18.92 5.21,21.72 4.83,22.1 v4.83,22.73
PARTICLE_A2  (via drill 0.2)
  Top 0.203: v3.43,23.5 3.56,23.62 8,23.62 8.42,23.2 U6.13
  Bottom 0.203: J2.10 1.27,10.16 2.54,11.43 2.54,13.46 2.92,13.84 2.92,15.11 3.3,15.49 3.3,17.53 4.83,19.05 4.83,21.59 4.06,22.35 4.06,22.86 v3.43,23.5
PARTICLE_A3  (via drill 0.2)
  Top 0.203: U6.14 7.92,23.07 7.75,23.24 3.94,23.24 v3.43,22.73
  Bottom 0.203: v3.43,22.73 3.43,22.35 4.45,21.34 4.45,19.18 2.92,17.65 2.92,15.62 2.54,15.24 2.54,13.97 1.27,12.7 J2.9
PARTICLE_A4  (via drill 0.2)
  Top 0.203: U6.19 4.24,20.78 v3.43,21.59
  Bottom 0.203: v3.43,21.59 4.06,20.95 4.06,19.3 2.54,17.78 2.54,15.75 J2.8
PARTICLE_A5  (via drill 0.2)
  Top 0.203: v3.45,20.78 3.95,20.28 U6.20
  Bottom 0.203: J2.7 3.68,19.43 3.68,20.55 v3.45,20.78
PARTICLE_D0  (via drill 0.2)
  Top 0.203: U6.57 14.86,18.28 14.22,17.65 v14.22,16.82
  Bottom 0.203: J3.1 16.26,7.11 16.26,9.78 16.64,10.16 16.64,10.79 16,11.43 16,14.22 14.73,15.49 14.73,16.31 v14.22,16.82
PARTICLE_D1  (via drill 0.2)
  Top 0.203: U6.58 14.47,18.78 v14.22,18.54
  Bottom 0.203: J3.2 18.8,6.86 17.53,8.13 17.53,9.91 17.02,10.41 17.02,10.92 16.38,11.56 16.38,14.61 15.11,15.88 15.11,16.76 14.22,17.65 v14.22,18.54
PARTICLE_D2  (via drill 0.2)
  Top 0.203: U6.56 15.5,17.78 v16,18.29
  Bottom 0.203: J3.3 16.76,11.68 16.76,16.15 16.51,16.41 16.51,16.74 16,17.25 v16,18.29
PARTICLE_D3  (via drill 0.2)
  Top 0.203: U6.55 16.27,17.28 v16.64,17.65
  Bottom 0.203: J3.4 19.05,12.7 17.78,13.97 17.78,17.27 17.4,17.65 v16.64,17.65 16.89,17.65
PARTICLE_D4
  Top 0.203: U6.59 15.77,19.28 17.78,17.27 17.78,16.51 19.05,15.24 J3.5
PARTICLE_D5
  Top 0.203: U6.60 15.78,19.78 18.54,17.02 J3.6
PARTICLE_D6  (via drill 0.2)
  Top 0.203: U6.48 14.46,13.51 v14.94,13.03
  Route2 0.203: J3.7 18.47,18.97 15.9,18.97 15.49,18.57 15.49,14.33 15.95,13.87 15.95,13.18 15.8,13.03 v14.94,13.03
PARTICLE_D7  (via drill 0.2)
  Top 0.203: U6.53 15.78,16.28 v16,16.51
  Bottom 0.203: v16,16.51 15.24,17.27 15.24,18.41 15.75,18.92 17.4,18.92 17.65,19.18 17.65,20.45 19.05,21.84 J3.8 18.8,22.1
PARTICLE_DAC  (via drill 0.2)
  Top 0.203: U6.21 3.33,19.78 2.74,20.37 v2.74,20.75
  Bottom 0.203: J2.6 2.46,20.75 v2.74,20.75
PARTICLE_RX  (via drill 0.2)
  Top 0.203: U6.62 16.05,20.78 v16.26,20.57
  Bottom 0.203: v16.26,20.57 16,20.83 14.22,20.83 12.7,22.35 6.6,22.35 5.59,23.37 4.57,23.37 3.81,24.13 3.05,24.13 2.39,23.47 1.67,23.47 1.27,23.88 J2.4
PARTICLE_TX  (via drill 0.2)
  Top 0.203: U6.63 15.95,21.28 v16.13,21.46
  Bottom 0.203: v16.13,21.46 14.1,21.46 12.83,22.73 6.73,22.73 5.71,23.75 4.7,23.75 3.43,25.02 2.67,25.02 2.29,25.4 2.29,26.16 J2.3
PARTICLE_WKP
  Top 0.203: 2.03,22.1 J2.5 1.27,21.29 2.54,20.02 2.54,19.56 2.79,19.3 6.12,19.3 U6.22
RED_LED  (via drill 0.2)
  Top 0.203: U6.40 10.42,12.32 v10.29,12.19 | v15.34,10.29 15.49,10.44 15.49,10.79 15.95,11.25 R1.1
  Bottom 0.203: v10.29,12.19 9.91,11.81 9.91,10.31 11.33,8.88 14.12,8.88 15.34,10.1 v15.34,10.29
SAM4L_SWDCLK  (via drill 0.2)
  Top 0.203: J4.4 5.97,6.99 6.48,7.49 6.48,8.51 7.37,9.4 v7.37,9.65 7.72,10.01 R12.1 | U6.9 10.42,22.09 10.92,21.59 v11.3,21.59
  Bottom 0.203: v7.37,9.65 7.37,11.43 8.51,12.57 9.27,12.57 9.78,13.08 10.79,13.08 11.18,13.46 11.18,14.48 11.68,14.99 12.95,16.26 12.95,19.94 v11.3,21.59
SAM4L_SWDIO  (via drill 0.2)
  Top 0.203: U6.10 9.92,21.83 v10.16,21.59 | J4.2 6.48,9.27 v6.48,9.65 6.71,9.88 R11.1
  Bottom 0.203: v6.48,9.65 6.99,10.16 6.99,11.56 8.51,13.08 9.14,13.08 9.65,13.59 10.41,13.59 10.79,13.97 10.79,14.61 10.16,15.24 9.4,15.24 8.51,16.13 8.51,19.94 v10.16,21.59
SAM4L_XIN1
  Top 0.203: U6.1 14.97,23.11 15.67,23.11 X2.3 16.76,23.73 C2.1
SAM4L_XOUT1
  Top 0.203: U6.2 13.92,23.06 14.22,23.37 14.22,25.07 X2.1 | 14.97,25.92 X2.1 | C3.1 13.54,26.42 14.37,26.42 X2.1
SENSORS_SCL  (via drill 0.2)
  Top 0.203: U3.5 4.32,13.41 4.01,13.72 3.73,13.72 3.59,13.86 3.59,14.59 3.71,14.71 4.12,14.71 v4.57,15.16 | v8.13,21.59 8.38,21.84 8.64,21.84 8.92,22.13 U6.12 8.92,23.21 8.13,24 4.79,24 U7.6 3.62,24.65 R8.1 | v14.73,31.5 14.61,31.38 U2.4
  Route15 0.203: v8.13,21.59 8.13,22.1 10.54,24.51 11.94,24.51 13.99,26.57 13.99,27.71 12.95,28.75 12.95,31.18 13.52,31.75 14.48,31.75 v14.73,31.5
  Bottom 0.203: v4.57,15.16 5.03,15.57 5.84,15.57 6.45,16.18 7.42,16.18 7.67,16.43 7.67,21.13 v8.13,21.59 | v14.73,31.5 14.73,31.7 TP7.TP
SENSORS_SDA  (via drill 0.2)
  Top 0.203: U3.6 3.23,13.71 3.23,14.69 4.18,15.63 | 4.18,15.63 4.29,15.75 4.83,15.75 5.31,15.27 v5.31,15.01 | v9.27,21.59 9.42,21.74 U6.11 9.42,23.22 8.26,24.38 7.31,24.38 U7.1 | R7.1 3.81,16 4.18,15.63 | v13.72,31.11 U2.6
  Route15 0.203: v9.27,21.59 9.27,22.75 10.65,24.13 13.16,24.13 14.68,25.65 14.68,27.86 13.72,28.83 v13.72,31.11
  Bottom 0.203: v5.31,15.01 5.99,15.01 6.73,15.75 7.52,15.75 8.05,16.28 8.05,20.37 v9.27,21.59 | v13.72,31.11 13.72,32.69 TP6.TP
VCC  (via drill 0.2)
  Top 0.203: U1.12 8.01,29.46 7.75,29.72 7.99,29.96 U1.11 8.26,30.09 v7.87,30.48 | U6.52 15.23,15.75 v16,15.75 | C20.1 v16,15.75 | v9.4,11.43 9.58,11.61 C19.1 9.58,12.5 9.92,12.84 U6.39 | U5.12 v16.84,9.48 16.84,9.68 C12.1 | D1.1 16.08,15.67 v16,15.75 | U6.61 15.78,20.28 16.26,19.81 16.76,19.81 | 16.76,19.81 17.09,20.14 C21.1 | 16.76,19.81 v17.02,19.56 | v4.83,10.87 4.52,10.87 3.7,10.05 3.7,8.75 J4.1 | U6.35 7.92,11.58 R12.2 R11.2 C14.1 5.33,11.38 v4.83,10.87 | v4.83,10.87 4.37,10.87 3.82,11.42 U3.1 | R9.2 5.08,14.22 v5.61,13.69 | 3.68,27.81 C24.1 3.23,27.41 R8.2 3.48,25.65 U7.5 | U6.8 10.92,23.37 v10.79,23.5 | v4.83,17.14 4.12,17.86 FB1.2 R7.2 | C17.1 R13.2 18.98,32.33 J3.12 18.14,32.26 17.53,31.64 | U2.1 17.53,31.64 | v9.91,4.45 10.14,4.68 U5.35 | v9.91,4.45 10.07,4.28 U5.36 | U2.14 17.15,28.33 17.53,28.7 17.53,31.64 | LED1.A 15.86,1.59 16.66,2.39 C11.1 | C6.1 10.03,4.32 v9.91,4.45 | v17.65,2.29 17.53,2.41 C11.1 | C11.1 16.84,2.59 U5.1 | v8.13,27.18 8.13,26.82 8.41,26.54 8.41,26.11 C13.1 | U1.20 11.43,27.33 v11.89,27.33
  Top 0.406: v3.81,29.97 3.93,29.85 U4.5 3.63,28.72 C24.1
  Route15 0.203: v16.84,9.48 16.81,9.48
  Bottom 0.203: v4.83,10.87 5.15,10.87 5.97,10.05 5.97,8.75 5.48,8.26 J5.1
  pour Route15: 9.27,0 9.27,5 0,5 0,36.58 20.32,36.58 20.32,3.05 18.8,0

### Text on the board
tPlace: RESET | B | SAM4L | Hail
bPlace: RESET BUTTON | USER BUTTON | SENSORS_SCL | SENSORS_SDA | FTDI_OUT | FTDI_IN | ACC_INT2 | !FTDI_RTS | NRF_RTS | ACC_INT1 | NRF_CTS | NRF_OUT | NRF_INT | !LIGHT_INT | NRF_IN | NRF JTAG | Ghena | B | Campbell | 03-2017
